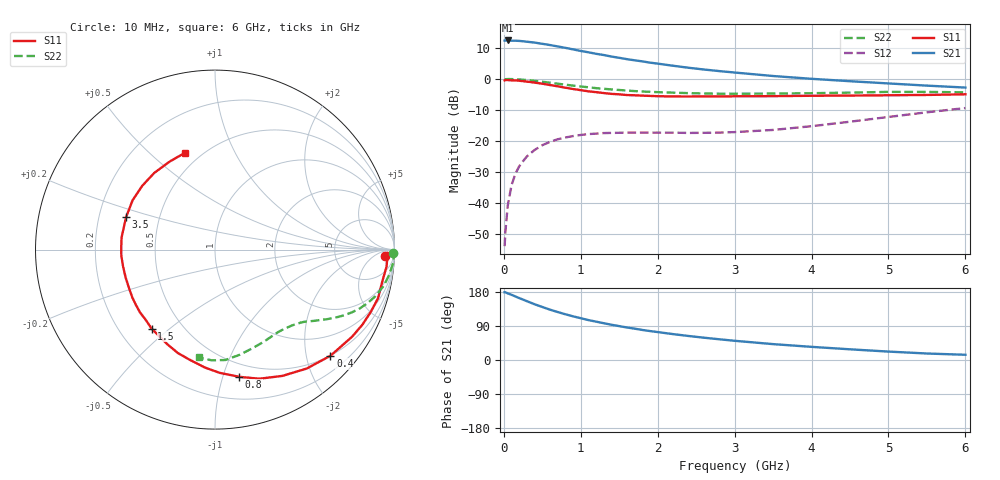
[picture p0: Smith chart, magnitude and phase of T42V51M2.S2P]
! Infineon Technologies  Discrete & RF Semiconductors
! BFR182T
! Si NPN RF Bipolar Junction Transistor in SC75
! VCE = 2.5 V  IC = 1.2 mA
! Common Emitter S-Parameters:  October  1999
# GHz  S  MA  R  50
!  f  S11  S21  S12  S22
! GHz  MAG  ANG  MAG  ANG  MAG  ANG  MAG  ANG
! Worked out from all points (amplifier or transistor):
!   36 points, 10 MHz to 6 GHz, reference 50 ohm
!   highest |S21| = 12.4 dB at 50 MHz (marker M1)
!   |S21| within 3 dB of that: start of sweep to 922.7 MHz
!   unconditionally stable (mu >= 1): 2.287 GHz to 4.517 GHz
!   at 250 MHz: K = 0.10, MSG = 19.3 dB, |S12| = -26.5 dB
!   at 1.4 GHz: K = 0.63, MSG = 12.3 dB, |S12| = -17.4 dB
!   at 6 GHz: K = 0.83, MSG = 3.3 dB, |S12| = -9.4 dB
!   S11 on the Smith chart (normalised r, x): 10 MHz: 25, -17; 400 MHz: 0.50, -2.48; 800 MHz: 0.38, -1.13; 1.5 GHz: 0.34, -0.44; 3.5 GHz: 0.32, +0.16; 6 GHz: 0.41, +0.66
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0.01  0.9476 -2.1  4.154 178.7  0.002 85.1  0.9912 -1.2
0.02  0.9627 -1.0  4.17 178.7  0.0034 98.2  0.9899 -0.8
0.05  0.9604 -5.6  4.179 175.9  0.0089 87.5  0.996 -2.2
0.1  0.9491 -10.7  4.149 172.1  0.0193 85.1  0.9951 -4.3
0.15  0.948 -16.6  4.138 167.7  0.0294 80.6  0.9863 -6.5
0.25  0.9219 -26.9  4.053 159.4  0.0471 74.7  0.9693 -10.5
0.4  0.8739 -42.6  3.862 147.1  0.0715 65.7  0.9307 -16.2
0.5  0.8371 -52.3  3.691 139.9  0.0852 60.8  0.9013 -19.3
0.6  0.7976 -61.9  3.523 132.8  0.0964 56.0  0.8697 -22.2
0.7  0.7607 -71.0  3.346 126.6  0.1063 52.2  0.838 -24.7
0.8  0.7217 -79.2  3.176 120.7  0.1134 48.2  0.808 -26.9
0.9  0.6873 -87.8  2.998 115.2  0.1197 45.2  0.78 -28.8
1.1  0.6302 -102.8  2.691 105.3  0.1288 40.2  0.7326 -32.0
1.3  0.5913 -116.4  2.431 97.0  0.1339 36.5  0.693 -34.7
1.5  0.5644 -128.7  2.193 89.4  0.1352 34.1  0.6633 -37.0
1.8  0.5373 -145.4  1.921 79.3  0.1364 32.3  0.6264 -40.5
2.2  0.5218 -162.3  1.633 68.3  0.1357 33.2  0.6007 -44.9
2.8  0.5227 178.0  1.339 54.7  0.1362 38.7  0.5782 -52.9
3.5  0.5275 160.0  1.115 41.9  0.1503 48.5  0.581 -62.2
4.5  0.539 139.0  0.919 28.2  0.2041 58.2  0.602 -76.9
5.5  0.5517 117.3  0.78 17.1  0.2895 58.8  0.6172 -91.7
6  0.5654 106.9  0.726 13.8  0.3392 56.0  0.6079 -98.6
